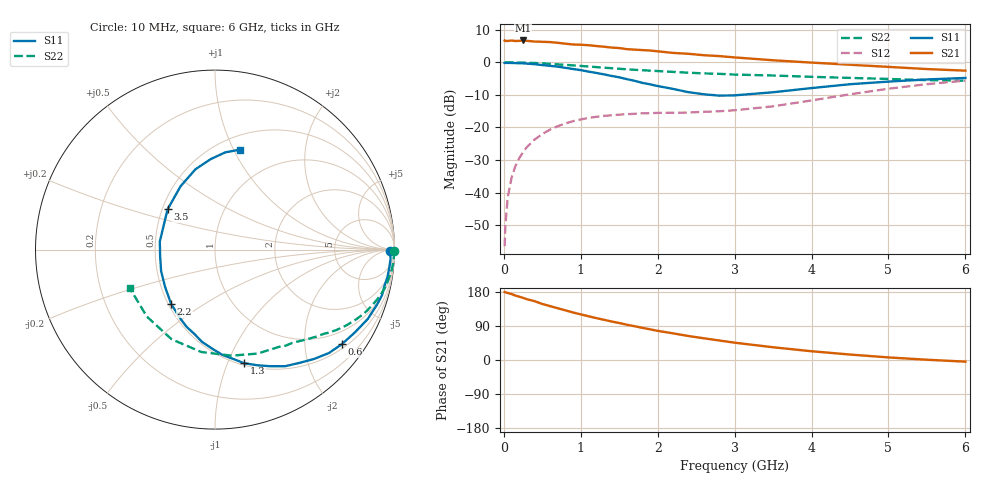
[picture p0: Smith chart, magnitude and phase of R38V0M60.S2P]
! SIEMENS Small Signal Semiconductors
! BFR181
! Si NPN RF Bipolar Junction Transistor in SOT23
! VCE = 8 V  IC = 0.6 mA
! Common Emitter S-Parameters:  May  1996
# GHz  S  MA  R  50
!  f  S11  S21  S12  S22
! GHz  MAG  ANG  MAG  ANG  MAG  ANG  MAG  ANG
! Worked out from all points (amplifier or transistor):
!   36 points, 10 MHz to 6 GHz, reference 50 ohm
!   highest |S21| = 6.7 dB at 250 MHz (marker M1)
!   |S21| within 3 dB of that: start of sweep to 1.833 GHz
!   unconditionally stable (mu >= 1): 2.323 GHz to 3.91 GHz
!   at 250 MHz: K = 0.13, MSG = 17.1 dB, |S12| = -27.6 dB
!   at 1.4 GHz: K = 0.63, MSG = 10.4 dB, |S12| = -16.3 dB
!   at 6 GHz: K = 0.90, MSG = 1.5 dB, |S12| = -5.6 dB
!   S11 on the Smith chart (normalised r, x): 10 MHz: 72, -33; 600 MHz: 0.61, -2.90; 1.3 GHz: 0.52, -1.15; 2.2 GHz: 0.52, -0.37; 3.5 GHz: 0.53, +0.27; 6 GHz: 0.64, +1.06
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0.01  0.9772 -0.6  2.159 179.7  0.0015 96.2  0.9998 -0.3
0.02  0.9769 -1.2  2.124 178.5  0.0031 80.5  0.9988 -0.7
0.05  0.9796 -3.2  2.127 176.9  0.0083 87.8  0.9973 -1.5
0.1  0.9762 -6.1  2.155 174.1  0.0168 87.3  0.9972 -2.9
0.15  0.9729 -9.1  2.123 170.1  0.0254 82.9  0.9948 -4.5
0.25  0.9644 -15.3  2.164 163.9  0.0418 79.0  0.9896 -7.4
0.4  0.935 -24.4  2.082 155.2  0.065 73.2  0.9754 -11.7
0.5  0.9063 -30.5  2.063 147.9  0.0791 69.3  0.9618 -14.3
0.6  0.8817 -36.7  2.044 142.2  0.0925 65.4  0.9462 -17.0
0.8  0.8217 -47.9  1.93 131.0  0.1149 58.4  0.9126 -21.9
1.1  0.7193 -64.6  1.829 115.5  0.1397 50.0  0.8616 -28.0
1.3  0.653 -75.7  1.735 106.2  0.1505 45.4  0.8268 -31.8
1.6  0.5505 -91.9  1.591 93.0  0.1598 40.6  0.7805 -36.5
1.8  0.483 -103.9  1.54 84.9  0.1648 38.8  0.7557 -39.1
2  0.4318 -116.2  1.474 76.9  0.1672 37.5  0.7338 -41.9
2.2  0.39 -128.7  1.393 70.3  0.1677 37.4  0.7116 -44.8
2.4  0.3474 -143.2  1.35 63.3  0.1692 38.2  0.6917 -47.6
2.8  0.3075 -174.1  1.245 51.5  0.1771 41.1  0.6645 -53.7
3.5  0.3465 139.7  1.074 33.6  0.2106 48.4  0.6265 -67.6
4.5  0.4604 103.7  0.917 14.4  0.3225 49.6  0.5756 -97.6
5.5  0.545 83.9  0.787 0.7  0.4613 37.5  0.5324 -135.6
6  0.5748 75.8  0.744 -4.4  0.5226 29.1  0.5207 -155.8
